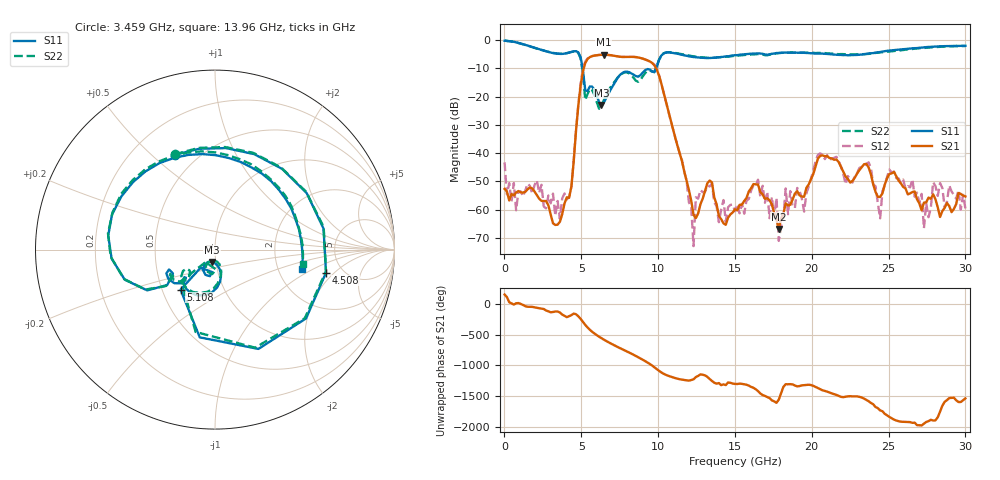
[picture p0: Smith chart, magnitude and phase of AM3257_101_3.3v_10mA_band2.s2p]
!Keysight Technologies,N5245B,MY58422270,A.16.20.02
!Date: Wednesday, June 18, 2025 22:52:47
!Correction: S11(C  2-Port  )
!S21(C  2-Port  )
!S12(C  2-Port  )
!S22(C  2-Port  )
!S2P File: Measurements: S11, S21, S12, S22:
# Hz S  dB  R 50
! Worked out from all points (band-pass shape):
!   201 points, 10 MHz to 30 GHz, reference 50 ohm
!   highest |S21| = -5.19 dB at 6.458 GHz (marker M1); lowest = -66.9 dB at 17.85 GHz (marker M2)
!   |S21| within 3 dB of the highest: 5.255 GHz to 9.627 GHz (4.372 GHz wide, 58.8 % of centre)
!   lowest |S11| = -23.0 dB at 6.308 GHz (marker M3), VSWR 1.15, Z = 47.9 - j6.66 ohm
!   |S11| at or under -10 dB: 5.088 GHz to 9.874 GHz (4.786 GHz wide, 64 % of centre)
!   |S22| runs from -24.3 to -0.1 dB; largest |S21 - S12| = 0.028
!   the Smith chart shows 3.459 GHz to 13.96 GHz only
!   S11 on the Smith chart (normalised r, x): 3.459 GHz: 0.38, +0.59; 4.508 GHz: 3.71, -1.58; 5.108 GHz: 0.62, -0.30; 13.96 GHz: 2.71, -0.76
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1e7  -0.25 -1.1  -52.65 154.1  -43.28 -52.5  -0.15 -1.6
1.2096e9  -1.47 -87.5  -53.95 -15.8  -55.29 9.5  -1.49 -87.2
3.45885e9  -4.83 113.0  -65.29 -121.9  -56.92 -109.2  -4.78 113.0
4.5085e9  -3.99 -11.7  -42.88 -155.9  -42.09 -141.0  -4.01 -11.0
5.1083e9  -10.63 -130.7  -11.05 68.9  -10.21 68.4  -11.78 -137.2
5.7081e9  -16.46 -110.8  -5.70 -92.0  -5.66 -93.2  -17.73 -109.9
6.3079e9  -22.95 -103.7  -5.21 164.1  -5.19 163.9  -23.51 -81.4
6.45785e9  -22.21 -88.6  -5.19 141.7  -5.18 141.5  -21.38 -72.9
7.35755e9  -13.48 -86.8  -5.78 21.3  -5.78 21.2  -13.34 -91.9
8.85705e9  -12.38 -134.0  -6.35 -167.5  -6.32 -167.4  -14.08 -134.6
1.005665e10  -7.12 -149.0  -12.53 -7.2  -12.31 -8.6  -7.00 -150.1
1.23059e10  -6.01 65.6  -61.80 -146.4  -72.90 -43.9  -5.74 67.0
1.275575e10  -6.24 42.9  -58.07 -66.2  -53.07 -99.4  -6.09 45.0
1.395535e10  -6.13 -12.4  -62.23 152.8  -64.43 -179.0  -6.08 -9.5
1.5005e10  -5.38 -52.6  -59.84 138.4  -60.57 152.4  -5.56 -49.8
1.65045e10  -4.71 -100.2  -51.12 21.7  -49.37 21.6  -4.97 -99.8
1.785405e10  -4.54 -133.4  -66.86 -116.9  -71.03 -89.1  -4.62 -133.5
2.01033e10  -4.74 162.1  -47.35 107.5  -46.13 113.4  -4.53 162.6
2.37021e10  -4.75 20.1  -45.06 -143.2  -43.25 -155.4  -4.89 26.3
2.445185e10  -4.20 -6.3  -55.49 67.4  -63.06 55.2  -4.38 -2.5
2.505165e10  -3.73 -25.7  -47.35 -39.1  -45.81 -40.9  -4.05 -23.7
3e10  -2.03 -124.6  -55.33 -96.9  -59.57 -37.6  -2.16 -126.1
